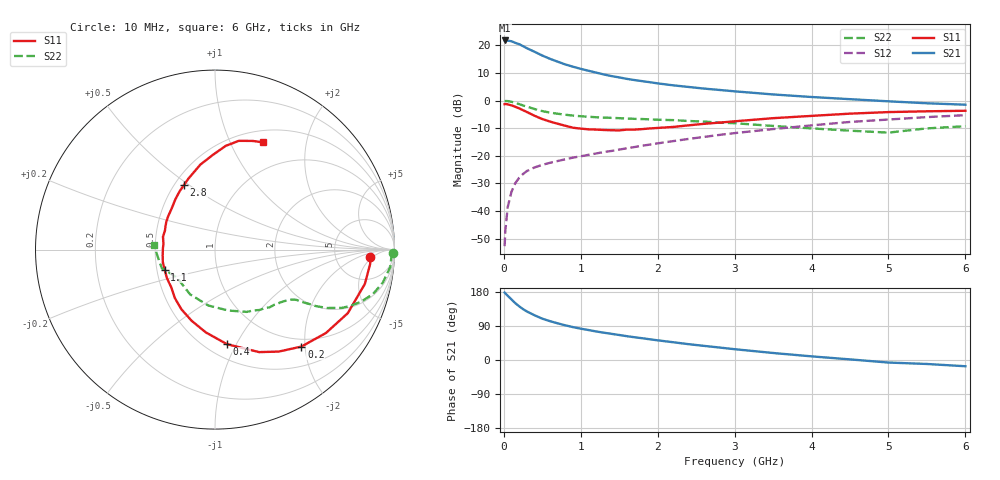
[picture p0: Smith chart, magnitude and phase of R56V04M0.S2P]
! SIEMENS Small Signal Semiconductors
! BFR183
! Si NPN RF Bipolar Junction Transistor in SOT23
! VCE = 6 V  IC = 4 mA
! Common Emitter S-Parameters:  May  1996
# GHz  S  MA  R  50
!  f  S11  S21  S12  S22
! GHz  MAG  ANG  MAG  ANG  MAG  ANG  MAG  ANG
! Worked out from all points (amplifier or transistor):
!   36 points, 10 MHz to 6 GHz, reference 50 ohm
!   highest |S21| = 21.8 dB at 10 MHz (marker M1)
!   |S21| within 3 dB of that: start of sweep to 313.9 MHz
!   unconditionally stable (mu >= 1): 1.17 GHz to 2.706 GHz
!   at 250 MHz: K = 0.36, MSG = 23.2 dB, |S12| = -26.6 dB
!   at 1.4 GHz: K = 1.06, MAG = 12.1 dB, |S12| = -18.2 dB
!   at 6 GHz: K = 0.88, MSG = 1.9 dB, |S12| = -5.3 dB
!   S11 on the Smith chart (normalised r, x): 10 MHz: 12, -4; 200 MHz: 0.85, -1.93; 400 MHz: 0.62, -0.92; 1.1 GHz: 0.55, -0.14; 2.8 GHz: 0.56, +0.48; 6 GHz: 0.64, +1.34
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0.01  0.8631 -2.6  12.33 178.0  0.0023 94.6  0.9915 -1.1
0.02  0.8684 -5.2  12.17 175.6  0.0045 85.7  0.9838 -2.3
0.05  0.8566 -12.9  12.26 169.6  0.0117 83.1  0.9812 -5.7
0.1  0.8202 -25.6  11.91 159.7  0.0224 77.3  0.9531 -11.1
0.15  0.7735 -36.9  11.14 149.8  0.0321 70.7  0.9144 -15.7
0.2  0.7236 -48.3  10.54 141.6  0.0401 66.5  0.8661 -19.5
0.25  0.67 -58.0  9.718 134.2  0.0468 62.5  0.8178 -22.5
0.3  0.6219 -66.7  8.911 128.0  0.053 59.9  0.7775 -24.7
0.4  0.5311 -82.8  7.68 117.9  0.0616 56.2  0.7045 -27.5
0.5  0.4642 -96.3  6.563 109.0  0.0685 54.1  0.6461 -29.2
0.6  0.4171 -108.3  5.728 102.5  0.0747 53.3  0.6063 -30.0
0.7  0.3815 -119.4  5.083 96.7  0.0805 53.1  0.5788 -30.7
0.9  0.3225 -138.8  4.117 86.7  0.0927 53.6  0.5362 -31.6
1.1  0.302 -158.3  3.482 79.1  0.1041 55.1  0.5105 -33.1
1.3  0.2936 -173.2  2.983 72.1  0.117 56.0  0.4925 -34.6
1.6  0.2985 166.1  2.479 62.8  0.137 56.7  0.474 -37.9
2.2  0.3333 136.3  1.895 46.9  0.1844 56.5  0.4433 -46.4
2.8  0.3994 115.7  1.563 33.0  0.2388 53.3  0.4 -58.0
3.5  0.4809 99.7  1.295 18.5  0.3051 46.9  0.3478 -77.5
4.5  0.581 84.1  1.063 1.6  0.4109 35.5  0.2854 -119.2
5.5  0.6407 70.9  0.896 -10.5  0.503 22.9  0.3141 -160.8
6  0.6553 65.7  0.844 -16.5  0.5455 14.6  0.3435 175.5
